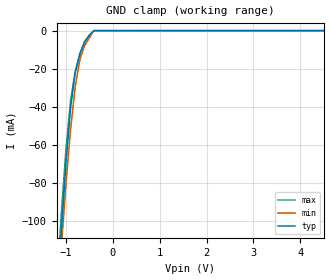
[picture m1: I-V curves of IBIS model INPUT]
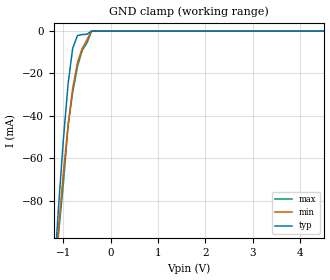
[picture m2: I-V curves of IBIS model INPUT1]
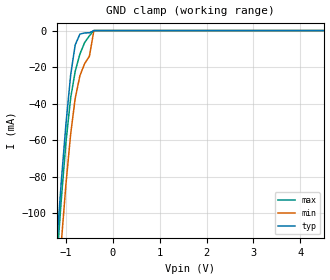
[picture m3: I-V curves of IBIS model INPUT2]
|   PERICOM SEMICONDUCTOR CORP
|   IBIS Model of PI6LC4833
|   Product Family: 6LC
|   56 Pin TQFN Package
[IBIS Ver] 3.2
[Comment char] |_char
[File Name] pi6lc4833zb.ibs
[File Rev] 2.0
[Source] File originated at Pericom Semiconductor Corp.
[Date] 09/12/11
[Disclaimer] (C) Copyright PERICOM Semiconductor Corporation
   All rights reserved
  Pericom Semiconductor Corporation hereby grants the user of
  this IBIS model a non-exclusive, nontransferable license to
  use this IBIS model under the following terms.
  This IBIS model is provided on an "AS IS" basis and Pericom
  makes absolutely no warranty with respect to the information
  contained herein. PERICOM DISCLAIMS AND CUSTOMER WAIVES ALL
  WARRANTIES, EXPRESSED OR IMPLIED, INCLUDING WARRANTIES OF
  MERCHANTABILITY OR FITNESS FOR A PARTICULAR PURPOSE. The
  entire risk as to quality and performance is with the customer.
  Accordingly, in no event shall the company be liable for any
  damages, whether in contract or tort, including any lost
  profits or other incidental, consequential, exemplary, or
  punitive damages arising out of the use or application of the
  IBIS model provided in this package. Further, Pericom reserves
  the right to make changes without notice to any product herein
  to improve reliability, function, or design. Pericom does not
  convey any license under patent rights or any other intellectual
  property rights, including those of third parties.
  The user is granted this license only to use the IBIS model
  and is not granted rights to sell, load, rent, lease or license
  the IBIS model in whole or in part, or in modified form to anyone
  other than user. User may modify the IBIS model to suit its specific
  application but rights to derivative works and such modifications
  shall belong to Pericom.
  Pericom is not obligated to provide maintenance or support
  for the licensed IBIS model.
  Contact Pericom at ATTN: APPLICATION ENGINEERING / IBIS MODELS
  3545 North First Street, San Jose, CA 95134
[Component] PI6LC4833zb
[Manufacturer] Pericom Semiconductor Corp.
[Package]
|   typ   min   max
R_pkg   3.400e-02   2.800e-02   3.900e-02
L_pkg   3.404e-09   2.704e-09   4.545e-09
C_pkg   4.280e-13   2.990e-13   5.710e-13
[Pin]   signal_name   model_name   R_pin   L_pin   C_pin
1   OC-B   INPUT   3.100e-02   2.704e-09   2.990e-13
2   FB0   INPUT   3.100e-02   2.704e-09   2.990e-13
3   VCCB   POWER   3.200e-02   2.990e-09   3.490e-13
4   VCCB   POWER   3.200e-02   2.990e-09   3.490e-13
| LVCMOS
5   QB0   OUTPUT1   3.200e-02   2.774e-09   3.180e-13
6   QB1   OUTPUT1   3.200e-02   2.774e-09   3.180e-13
7   VDD_OSC   POWER   3.200e-02   2.990e-09   3.490e-13
8   X1   INPUT2   3.100e-02   2.704e-09   2.990e-13
9   X2   OUTPUT1   3.200e-02   2.774e-09   3.180e-13
10   IN+   INPUT1   3.100e-02   2.704e-09   2.990e-13
11   IN-   INPUT1   3.100e-02   2.704e-09   2.990e-13
12   IN_Sel   INPUT   3.500e-02   3.598e-09   4.890e-13
13   OC-R   INPUT   3.500e-02   3.598e-09   4.890e-13
14   Sel_Freq2  INPUT   3.500e-02   3.598e-09   4.890e-13
15   VccR   POWER   3.200e-02   2.990e-09   3.490e-13
16   Qref0   OUTPUT1   3.500e-02   3.598e-09   4.890e-13
17   Qref1   OUTPUT1   3.500e-02   3.598e-09   4.890e-13
18   Qref2   OUTPUT1   3.500e-02   3.598e-09   4.890e-13
19   VccR   POWER   3.200e-02   2.990e-09   3.490e-13
20   GND   GND   3.900e-02   4.133e-09   5.710e-13
21   VDDA2   POWER   3.200e-02   2.990e-09   3.490e-13
22   VDD_PLL2   POWER   3.200e-02   2.990e-09   3.490e-13
| LVPECL
23   QD0+   OUTPUT2   3.200e-02   2.990e-09   3.490e-13
24   QD0-   OUTPUT2   3.200e-02   2.990e-09   3.490e-13
25   Sel_Freq2  INPUT   3.500e-02   3.598e-09   4.890e-13
| LVCMOS
26   QD1   OUTPUT1   3.200e-02   2.990e-09   3.490e-13
27   QD2   OUTPUT1   3.200e-02   2.990e-09   3.490e-13
28   VccD   POWER   3.200e-02   2.990e-09   3.490e-13
29   OC-C   INPUT   3.100e-02   2.704e-09   2.990e-13
30   Sel_Freq3  INPUT   3.500e-02   3.598e-09   4.890e-13
| LVPECL
31   QC0+   OUTPUT2   3.200e-02   2.990e-09   3.490e-13
32   QC0-   OUTPUT2   3.200e-02   2.990e-09   3.490e-13
33   VccC0   POWER   3.200e-02   2.990e-09   3.490e-13
| LVCMOS
34   QC1   OUTPUT1   3.500e-02   3.598e-09   4.890e-13
35   VccC1   POWER   3.200e-02   2.990e-09   3.490e-13
36   VCCA   POWER   3.200e-02   2.990e-09   3.490e-13
37   PLL_BYPS   INPUT   3.100e-02   2.704e-09   2.990e-13
38   SS0   INPUT   3.100e-02   2.704e-09   2.990e-13
39   SS1   INPUT   3.100e-02   2.704e-09   2.990e-13
40   OC-A   INPUT   3.100e-02   2.704e-09   2.990e-13
41   FA0   INPUT   3.100e-02   2.704e-09   2.990e-13
42   FA1   INPUT   3.100e-02   2.704e-09   2.990e-13
43   IREF   OUTPUT1   3.500e-02   3.598e-09   4.890e-13
| HCSL
44   QA0+   OUTPUT3   3.200e-02   2.990e-09   3.490e-13
45   QA0-   OUTPUT3   3.200e-02   2.990e-09   3.490e-13
46   VccA   POWER   3.200e-02   2.990e-09   3.490e-13
47   QA1+   OUTPUT3   3.200e-02   2.990e-09   3.490e-13
48   QA1-   OUTPUT3   3.200e-02   2.990e-09   3.490e-13
49   GND   GND   3.900e-02   4.133e-09   5.710e-13
50   QA2+   OUTPUT3   3.200e-02   2.990e-09   3.490e-13
51   QA2-   OUTPUT3   3.200e-02   2.990e-09   3.490e-13
52   VccA   POWER   3.200e-02   2.990e-09   3.490e-13
53   QA3+   OUTPUT3   3.200e-02   2.990e-09   3.490e-13
54   QA3-   OUTPUT3   3.200e-02   2.990e-09   3.490e-13
55   GND   GND   3.900e-02   4.133e-09   5.710e-13
56   VDDA1   POWER   3.200e-02   2.990e-09   3.490e-13
[Diff Pin] inv_pin  vdiff   tdelay_typ  tdelay_min   tdelay_max
| LVPECL
23   24   NA   0ns   -0.05ns   0.05ns
31   32   NA   0ns   -0.05ns   0.05ns
| HCSL
44   45   NA   0ns   -0.05ns   0.05ns
47   48   NA   0ns   -0.05ns   0.05ns
50   51   NA   0ns   -0.05ns   0.05ns
53   54   NA   0ns   -0.05ns   0.05ns
| Models and submodels in the file (6): INPUT (Input), INPUT1 (Input), INPUT2 (Input), OUTPUT1 (Output), OUTPUT2 (Output_ECL), OUTPUT3 (Output)
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|   Model INPUT (CMOS)
[Model] INPUT
Model_type Input
Vinl = 800mV
Vinh = 2.00V
| variable   typ   min   max
C_comp   4.00pF   3.8pF   4.2pF
[Voltage Range]   3.30V   3.135V   3.465V
[GND Clamp Reference]   0.00V   0.00V   0.00V
[POWER Clamp Reference]  3.30V   3.135V   3.465V
[temperature range]   25   70   -20
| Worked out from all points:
|   GND clamp passes 1 mA (typ) near -0.44 V on its own axis
[GND Clamp]
| Voltage   I(typ)   I(min)   I(max)
-3.3V     -1.197A    -928.6mA   -1.231A
-1.202V   -148.7mA   -152.6mA   -137.9mA
-1.101V   -107.3mA   -115.3mA   -97.36mA
-999.4mV  -69.97mA   -80.92mA   -62.79mA
-898.4mV  -40.31mA   -51.53mA   -36.54mA
-802.2mV  -22.43mA   -29.68mA   -21.51mA
-701mV    -12.09mA   -15.2mA    -12.13mA
-599.9mV  -5.88mA    -7.79mA    -5.84mA
-498.6mV  -2.39mA    -3.78mA    -2.44mA
-402.8mV  0A         0A         0A
6.601V    30uA       0A         0A
[POWER Clamp]   |Note: Vtable = Vcc - Voutput
| Voltage   I(typ)   I(min)   I(max)
-3.3V     0A         0A         0A
0V        0A         0A         0A
|   Model INPUT1 (Diff. input)
[Model] INPUT1
Model_type Input
Vinl = 800mV
Vinh = 2.00V
| variable   typ   min   max
C_comp   4.00pF   3.8pF   4.2pF
[Voltage Range]   3.30V   3.135V   3.465V
[GND Clamp Reference]   0.00V   0.00V   0.00V
[POWER Clamp Reference]  3.30V   3.135V   3.465V
[temperature range]   25   70   -20
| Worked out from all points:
|   GND clamp passes 1 mA (typ) near -0.47 V on its own axis
[GND Clamp]
| Voltage   I(typ)   I(min)  I(max)
-3.3V     -941.9mA   -788.4mA   -855.5mA
-1.202V   -118.1mA   -121.6mA   -132.7mA
-1.101V   -82.96mA   -93.49mA   -95.47mA
-999.4mV  -51.56mA   -67.1mA    -72.17mA
-898.3mV  -24.83mA   -44.37mA   -44.54mA
-802.1mV  -8.16mA    -26.98mA   -28.85mA
-700.9mV  -2.12mA    -14.93mA   -16.82mA
-599.8mV  -1.62mA    -8.15mA    -9.03mA
-498.5mV  -1.48mA    -4.01mA    -5.54mA
-402.9mV  0A         0A         0A
6.602V    0A         0A         0A
[POWER Clamp]   |Note: Vtable = Vcc - Voutput
| Voltage   I(typ)   I(min)   I(max)
-3.3V     0A         0A         0A
0V        0A         0A         0A
|   Model INPUT2
[Model] INPUT2
Model_type Input
Vinl = 0.80V
Vinh = 2.00V
| variable   typ   min   max
C_comp   4.00pF   3.8pF   4.2pF
[Voltage Range]   3.30V   3.135V   3.465V
[GND Clamp Reference]   0.00V   0.00V   0.00V
[POWER Clamp Reference]  3.30V   3.135V   3.465V
[temperature range]   25   70   -20
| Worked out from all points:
|   GND clamp passes 1 mA (typ) near -0.48 V on its own axis
[GND Clamp]
| Voltage   I(typ)   I(min)   I(max)
-3.3V     -916.6mA   -1.057A    -1.075A
-1.202V   -119.6mA   -152.7mA   -129.7mA
-1.101V   -83.43mA   -117.1mA   -93.38mA
-999.5mV  -51.29mA   -84.23mA   -61.35mA
-898.4mV  -24.31mA   -56.66mA   -36.88mA
-802.3mV  -7.88mA    -37.26mA   -22.34mA
-701.1mV  -1.92mA    -24.67mA   -12.83mA
-599.9mV  -1.27mA    -18.1mA    -6.55mA
-498.7mV  -1.22mA    -14.03mA   -2.87mA
-403mV    0A         0A         0A
6.602V    0A         0A         0A
[POWER Clamp]   |Note: Vtable = Vcc - Voutput
| Voltage   I(typ)   I(min)   I(max)
-3.3V     0A         0A         0A
0V        0A         0A         0A
